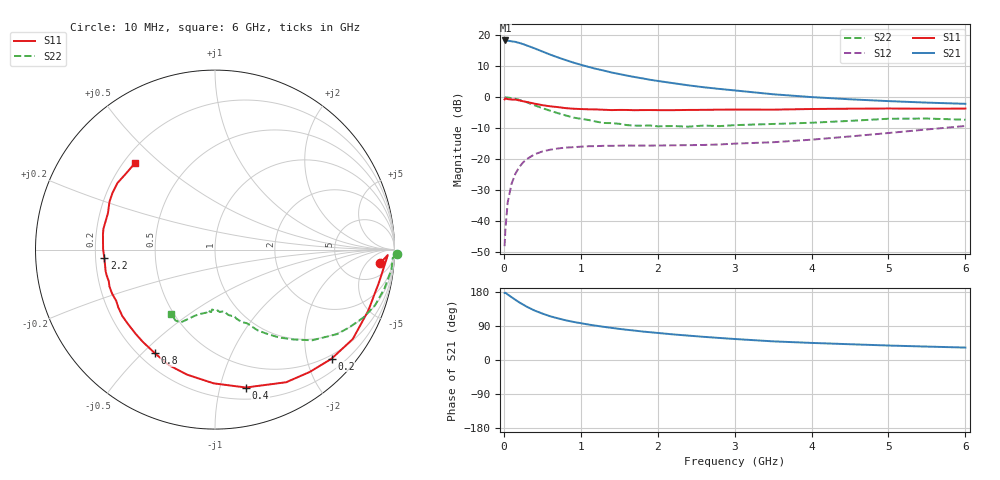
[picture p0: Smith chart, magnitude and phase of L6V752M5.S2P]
!  INFINEON TECHNOLOGIES Small Signal Semiconductors
! BFR380L3 , Si-NPN RF-Transistor in TSLP-3-1
!  Vce=0.75 V,  Ic=2.5 mA
! Common Emitter S-Parameters:  07. March 2005
#  GHz  S  MA  R  50
! f  S11  S21  S12  S22
! GHz  Mag  Ang  Mag  Ang  Mag  Ang  Mag  Ang
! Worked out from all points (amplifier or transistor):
!   36 points, 10 MHz to 6 GHz, reference 50 ohm
!   highest |S21| = 18.4 dB at 20 MHz (marker M1)
!   |S21| within 3 dB of that: start of sweep to 444 MHz
!   unconditionally stable (mu >= 1): 2.598 GHz to 4.884 GHz
!   at 250 MHz: K = 0.11, MSG = 19.1 dB, |S12| = -21.1 dB
!   at 1.4 GHz: K = 0.62, MSG = 11.9 dB, |S12| = -15.7 dB
!   at 6 GHz: K = 0.96, MSG = 3.6 dB, |S12| = -9.3 dB
!   S11 on the Smith chart (normalised r, x): 10 MHz: 12, -13; 200 MHz: 0.42, -2.47; 400 MHz: 0.30, -1.20; 800 MHz: 0.26, -0.54; 2.2 GHz: 0.24, -0.03; 6 GHz: 0.24, +0.41
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0.01  0.9236 -4.6  8.247 177.0  0.0039 84.7  1.013 -1.4
0.02  0.9634 -1.8  8.293 177.5  0.0072 93.8  0.991 -2.7
0.05  0.9321 -11.2  8.209 172.8  0.0199 84.4  0.9893 -6.5
0.1  0.9192 -21.8  8.039 165.9  0.0397 78.3  0.9685 -13.0
0.15  0.9151 -33.0  7.87 158.8  0.0579 72.0  0.9437 -19.3
0.2  0.8896 -43.1  7.571 152.1  0.074 67.0  0.9092 -24.6
0.3  0.8386 -61.8  6.868 140.4  0.1002 57.6  0.8272 -34.7
0.4  0.7873 -77.4  6.175 130.5  0.1196 50.0  0.7408 -43.0
0.5  0.7452 -90.6  5.506 122.6  0.1325 44.4  0.667 -48.7
0.6  0.7139 -102.6  4.91 115.5  0.1416 39.7  0.6062 -53.9
0.7  0.6931 -111.8  4.422 110.1  0.1482 37.0  0.5541 -58.1
0.8  0.6673 -120.2  4.009 105.0  0.1534 34.0  0.5097 -62.1
0.9  0.6526 -128.1  3.65 100.7  0.1556 32.1  0.4698 -64.8
1.1  0.638 -139.3  3.101 93.5  0.1614 30.0  0.4288 -69.9
1.5  0.6236 -156.9  2.376 82.1  0.1646 28.3  0.3723 -78.3
1.9  0.6213 -168.8  1.919 73.3  0.165 29.4  0.3486 -85.8
2.2  0.6185 -175.8  1.69 67.6  0.167 31.4  0.3423 -88.3
2.8  0.63 172.2  1.365 58.2  0.1721 37.8  0.3411 -97.1
3.5  0.6302 161.1  1.118 49.2  0.1872 44.8  0.3697 -103.6
4.5  0.6527 151.0  0.927 41.6  0.2323 54.8  0.4149 -111.2
5.5  0.6524 139.6  0.819 35.4  0.3014 58.6  0.4521 -119.2
6  0.6562 133.0  0.783 32.8  0.3428 58.4  0.433 -124.3
